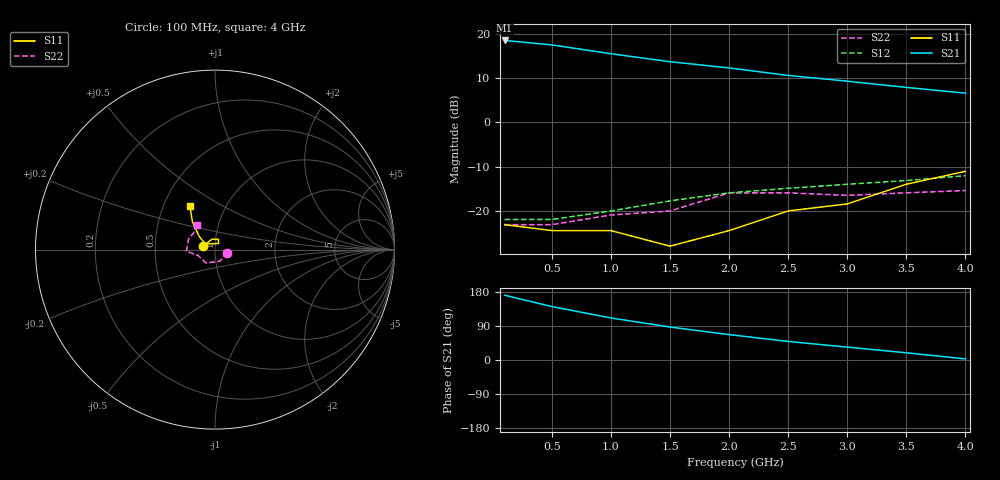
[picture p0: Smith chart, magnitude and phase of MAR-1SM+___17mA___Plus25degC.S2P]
! Mini-Circuits
! S2P DATA File Format
! Type: MMIC Amplifier
! Model: MAR-1SM+
! TEST CONDITIONS: Icc = 17mA @Temperature = +25degC
! S Parameters are in dB deg format
# MHz S DB R 50
!  FREQ  dB(S11)  PHS(S11)  dB(S21)  PHS(S21)  dB(S12)  PHS(S12)  dB(S22)  PHS(S22)
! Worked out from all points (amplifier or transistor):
!   9 points, 100 MHz to 4 GHz, reference 50 ohm
!   highest |S21| = 18.5 dB at 100 MHz (marker M1)
!   |S21| within 3 dB of that: start of sweep to 1 GHz
!   unconditionally stable (mu >= 1): start of sweep to end of sweep
!   at 500 MHz: K = 1.13, MAG = 17.5 dB, |S12| = -21.9 dB
!   at 2 GHz: K = 1.07, MAG = 12.5 dB, |S12| = -15.9 dB
!   at 4 GHz: K = 1.12, MAG = 7.2 dB, |S12| = -12.0 dB
100  -23.10 164.0  18.50 171.0  -21.94 4.0  -23.10 -14.0
500  -24.44 106.0  17.50 141.0  -21.94 15.0  -23.10 -68.0
1000  -24.44 72.0  15.50 111.0  -20.00 24.0  -20.92 -124.0
1500  -27.96 59.0  13.70 87.0  -17.72 26.0  -20.00 -161.0
2000  -24.44 149.0  12.30 67.0  -15.92 21.0  -15.92 -177.0
2500  -20.00 142.0  10.60 49.0  -14.89 18.0  -15.92 155.0
3000  -18.42 139.0  9.30 34.0  -13.98 12.0  -16.48 144.0
3500  -13.97 129.0  7.90 19.0  -13.15 5.0  -15.92 135.0
4000  -11.06 120.0  6.60 3.0  -12.04 -4.0  -15.39 127.0
